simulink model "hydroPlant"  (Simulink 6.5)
settings: Solver=ode23tb  StartTime=0.0  StopTime=10000  MaxStep=0.5  RelTol=1e-3
undefined symbols (not defined in the file or in its folder): Hydorplant_sf

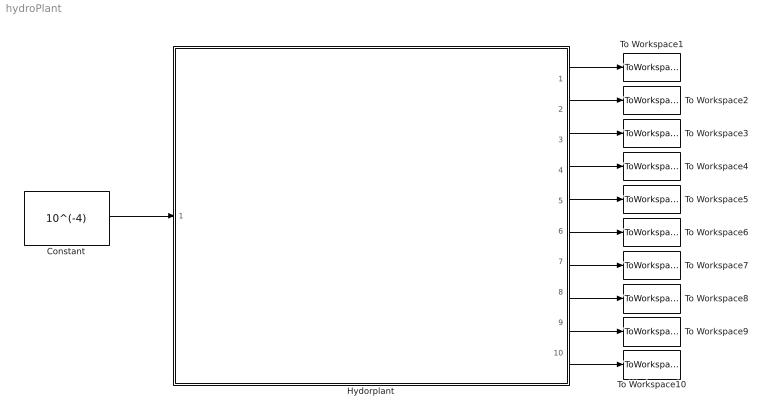
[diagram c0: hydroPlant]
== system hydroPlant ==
  Constant : Constant  Value=10^(-4)  OutDataType=sfix(16)  ConRadixGroup=Use specified scaling  OutScaling=2^0  SampleTime=inf  FramePeriod=inf
  Hydorplant : Subsystem
  To Workspace1 : ToWorkspace  VariableName=time  SampleTime=-1  SaveFormat=Array
  To Workspace10 : ToWorkspace  VariableName=P  SampleTime=-1  SaveFormat=Array
  To Workspace2 : ToWorkspace  VariableName=x  SampleTime=-1  SaveFormat=Array
  To Workspace3 : ToWorkspace  VariableName=h_W  SampleTime=-1  SaveFormat=Array
  To Workspace4 : ToWorkspace  VariableName=p_F  SampleTime=-1  SaveFormat=Array
  To Workspace5 : ToWorkspace  VariableName=V_flw_T  SampleTime=-1  SaveFormat=Array
  To Workspace6 : ToWorkspace  VariableName=V_flw_F  SampleTime=-1  SaveFormat=Array
  To Workspace7 : ToWorkspace  VariableName=omega  SampleTime=-1  SaveFormat=Array
  To Workspace8 : ToWorkspace  VariableName=U  SampleTime=-1  SaveFormat=Array
  To Workspace9 : ToWorkspace  VariableName=I  SampleTime=-1  SaveFormat=Array
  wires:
  Hydorplant/1(time) -> To Workspace1/1
  Hydorplant/2(x) -> To Workspace2/1
  Hydorplant/3(h_W) -> To Workspace3/1
  Hydorplant/4(p_F) -> To Workspace4/1
  Hydorplant/5(v_flw_T) -> To Workspace5/1
  Hydorplant/6(v_flw_F) -> To Workspace6/1
  Hydorplant/7(omega) -> To Workspace7/1
  Hydorplant/8(U) -> To Workspace8/1
  Hydorplant/9(I) -> To Workspace9/1
  Hydorplant/10(P) -> To Workspace10/1
  Constant/1 -> Hydorplant/1(u)

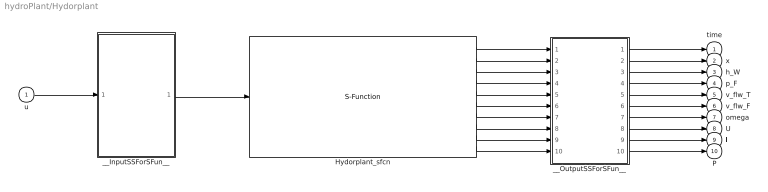
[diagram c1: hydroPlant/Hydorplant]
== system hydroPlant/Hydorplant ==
  u : Inport
  Hydorplant_sfcn : S-Function  FunctionName=Hydorplant_sf  SFunctionModules=""  mask{rtw_sf_name=Hydorplant_sf, showVar=off}
      mask prompts: rtw_sf_name "Generated S-function name (model_sf):"; showVar "Show module list"
      mask help: Real-Time Workshop generated S-function.
      mask init:
      | displist = '';
      | if ~strcmp(get_param(gcb, 'FunctionName'), rtw_sf_name);
      |   set_param(gcb, 'FunctionName', rtw_sf_name);
      | end
      | % Check if we are generating RTW code
      | rtw_mode = false;
      | if strcmpi(get_param(bdroot(gcb),'SimulationStatus'),'Initializing')
      | 	rtw_mode = strcmpi(get_param(bdroot(gcb),'BuildingRTWCode'),'on') && ...
      | 		~strcmpi(get_param(bdroot(gcb),'TargetStyle'),'SimulationTarget');
      | end
      | if showVar || rtw_mode
      | 	if exist('rtwsfunc') == 2 | exist('rtwsfunc') == 6
      | 		tmplist = rtwsfunc(rtw_sf_name,gcb);
      | 		tmplist = ['\nList of Modules:\n', tmplist];
      | 	elseif showVar
      | 		tmplist = '\nList of Modules:\nRTW not licensed\n';
      |  	end
      | end
      | if showVar
      |   displist = tmplist;
      | end
  __InputSSForSFun__ : Subsystem
  __OutputSSForSFun__ : Subsystem
  time : Outport  PortDimensions=1  SampleTime=[-1 0]  DataType=double
  x : Outport  Port=2  PortDimensions=1  SampleTime=[-1 0]  DataType=double
  h_W : Outport  Port=3  PortDimensions=1  SampleTime=[-1 0]  DataType=double
  p_F : Outport  Port=4  PortDimensions=1  SampleTime=[-1 0]  DataType=double
  v_flw_T : Outport  Port=5  PortDimensions=1  SampleTime=[-1 0]  DataType=double
  v_flw_F : Outport  Port=6  PortDimensions=1  SampleTime=[-1 0]  DataType=double
  omega : Outport  Port=7  PortDimensions=1  SampleTime=[-1 0]  DataType=double
  U : Outport  Port=8  PortDimensions=1  SampleTime=[-1 0]  DataType=double
  I : Outport  Port=9  PortDimensions=1  SampleTime=[-1 0]  DataType=double
  P : Outport  Port=10  PortDimensions=1  SampleTime=[-1 0]  DataType=double
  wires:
  u/1 -> __InputSSForSFun__/1(u)
  __InputSSForSFun__/1(__UniqueOutportName__1__) -> Hydorplant_sfcn/1
  Hydorplant_sfcn/1 -> __OutputSSForSFun__/1(__UniqueInportName__1__)
  Hydorplant_sfcn/2 -> __OutputSSForSFun__/2(__UniqueInportName__2__)
  Hydorplant_sfcn/3 -> __OutputSSForSFun__/3(__UniqueInportName__3__)
  Hydorplant_sfcn/4 -> __OutputSSForSFun__/4(__UniqueInportName__4__)
  Hydorplant_sfcn/5 -> __OutputSSForSFun__/5(__UniqueInportName__5__)
  Hydorplant_sfcn/6 -> __OutputSSForSFun__/6(__UniqueInportName__6__)
  Hydorplant_sfcn/7 -> __OutputSSForSFun__/7(__UniqueInportName__7__)
  Hydorplant_sfcn/8 -> __OutputSSForSFun__/8(__UniqueInportName__8__)
  Hydorplant_sfcn/9 -> __OutputSSForSFun__/9(__UniqueInportName__9__)
  Hydorplant_sfcn/10 -> __OutputSSForSFun__/10(__UniqueInportName__10__)
  __OutputSSForSFun__/1(time) -> time/1
  __OutputSSForSFun__/2(x) -> x/1
  __OutputSSForSFun__/3(h_W) -> h_W/1
  __OutputSSForSFun__/4(p_F) -> p_F/1
  __OutputSSForSFun__/5(v_flw_T) -> v_flw_T/1
  __OutputSSForSFun__/6(v_flw_F) -> v_flw_F/1
  __OutputSSForSFun__/7(omega) -> omega/1
  __OutputSSForSFun__/8(U) -> U/1
  __OutputSSForSFun__/9(I) -> I/1
  __OutputSSForSFun__/10(P) -> P/1

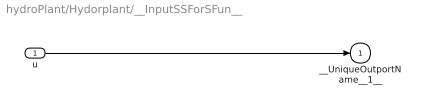
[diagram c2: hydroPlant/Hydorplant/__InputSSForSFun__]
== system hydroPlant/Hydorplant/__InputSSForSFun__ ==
  u : Inport
  __UniqueOutportName__1__ : Outport
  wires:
  u/1 -> __UniqueOutportName__1__/1

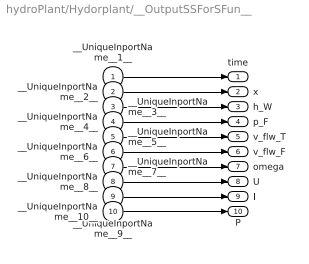
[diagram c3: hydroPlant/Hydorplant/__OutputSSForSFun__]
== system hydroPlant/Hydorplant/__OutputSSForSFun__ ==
  __UniqueInportName__1__ : Inport
  __UniqueInportName__2__ : Inport  Port=2
  __UniqueInportName__3__ : Inport  Port=3
  __UniqueInportName__4__ : Inport  Port=4
  __UniqueInportName__5__ : Inport  Port=5
  __UniqueInportName__6__ : Inport  Port=6
  __UniqueInportName__7__ : Inport  Port=7
  __UniqueInportName__8__ : Inport  Port=8
  __UniqueInportName__9__ : Inport  Port=9
  __UniqueInportName__10__ : Inport  Port=10
  time : Outport  PortDimensions=1  SampleTime=[-1 0]  DataType=double
  x : Outport  Port=2  PortDimensions=1  SampleTime=[-1 0]  DataType=double
  h_W : Outport  Port=3  PortDimensions=1  SampleTime=[-1 0]  DataType=double
  p_F : Outport  Port=4  PortDimensions=1  SampleTime=[-1 0]  DataType=double
  v_flw_T : Outport  Port=5  PortDimensions=1  SampleTime=[-1 0]  DataType=double
  v_flw_F : Outport  Port=6  PortDimensions=1  SampleTime=[-1 0]  DataType=double
  omega : Outport  Port=7  PortDimensions=1  SampleTime=[-1 0]  DataType=double
  U : Outport  Port=8  PortDimensions=1  SampleTime=[-1 0]  DataType=double
  I : Outport  Port=9  PortDimensions=1  SampleTime=[-1 0]  DataType=double
  P : Outport  Port=10  PortDimensions=1  SampleTime=[-1 0]  DataType=double
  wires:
  __UniqueInportName__1__/1 -> time/1
  __UniqueInportName__2__/1 -> x/1
  __UniqueInportName__3__/1 -> h_W/1
  __UniqueInportName__4__/1 -> p_F/1
  __UniqueInportName__5__/1 -> v_flw_T/1
  __UniqueInportName__6__/1 -> v_flw_F/1
  __UniqueInportName__7__/1 -> omega/1
  __UniqueInportName__8__/1 -> U/1
  __UniqueInportName__9__/1 -> I/1
  __UniqueInportName__10__/1 -> P/1
